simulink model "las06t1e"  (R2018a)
settings: Solver=ode45  StartTime=0.0  StopTime=50  MaxStep=10  MinStep=0.0001  RelTol=1e-3  AbsTol=1e-3  EnableMultiTasking=on
undefined symbols (not defined in the file or in its folder): omega, ts

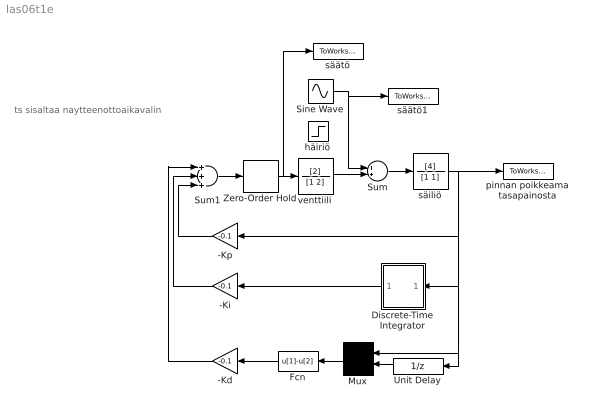
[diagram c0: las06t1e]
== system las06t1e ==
  note: ts sisaltaa naytteenottoaikavalin
  -Kd : Gain  Gain=-0.1
  -Ki : Gain  Gain=-0.1
  -Kp : Gain  Gain=-0.1
  Discrete-Time Integrator : Subsystem  mask(Discrete-Time Integrator){X0=0, Ts=ts}
      mask prompts: X0 "Initial Condition:"; Ts "Sample Time:"
      mask help: Discrete-Time Integrator:
  Fcn : Fcn  Expr=u[1]-u[2]
  Mux : Mux  Inputs=2
  Sine Wave : Sin  Frequency=omega  SampleTime=0
  Sum : Sum
  Sum1 : Sum  Inputs=+++
  Unit Delay : UnitDelay  SampleTime=ts
  Zero-Order Hold : ZeroOrderHold  SampleTime=ts
  häiriö : Step  Time=3  After=-1
  pinnan poikkeama tasapainosta : ToWorkspace  VariableName=y
  säiliö : TransferFcn  Numerator=[4]  Denominator=[1 1]
  säätö : ToWorkspace  VariableName=u
  säätö1 : ToWorkspace  VariableName=vaw  SampleTime=-1
  venttiili : TransferFcn  Numerator=[2]  Denominator=[1 2]
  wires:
  venttiili/1 -> Sum/2
  Sum/1 -> säiliö/1
  säiliö/1 -> pinnan poikkeama tasapainosta/1, -Kp/1, Unit Delay/1, Mux/1, Discrete-Time Integrator/1(in_1)
  -Kp/1 -> Sum1/3
  Mux/1 -> Fcn/1
  Unit Delay/1 -> Mux/2
  Fcn/1 -> -Kd/1
  Discrete-Time Integrator/1(out_1) -> -Ki/1
  Zero-Order Hold/1 -> venttiili/1, säätö/1
  Sum1/1 -> Zero-Order Hold/1
  -Ki/1 -> Sum1/2
  -Kd/1 -> Sum1/1
  Sine Wave/1 -> Sum/1, säätö1/1

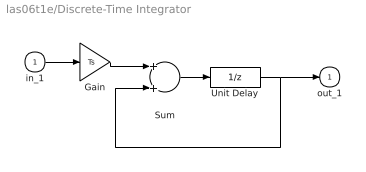
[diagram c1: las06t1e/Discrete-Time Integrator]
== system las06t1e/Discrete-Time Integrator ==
  in_1 : Inport
  Gain : Gain  Gain=Ts
  Sum : Sum
  Unit Delay : UnitDelay  InitialCondition=X0  SampleTime=Ts
  out_1 : Outport
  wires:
  Gain/1 -> Sum/1
  in_1/1 -> Gain/1
  Sum/1 -> Unit Delay/1
  Unit Delay/1 -> out_1/1, Sum/2
